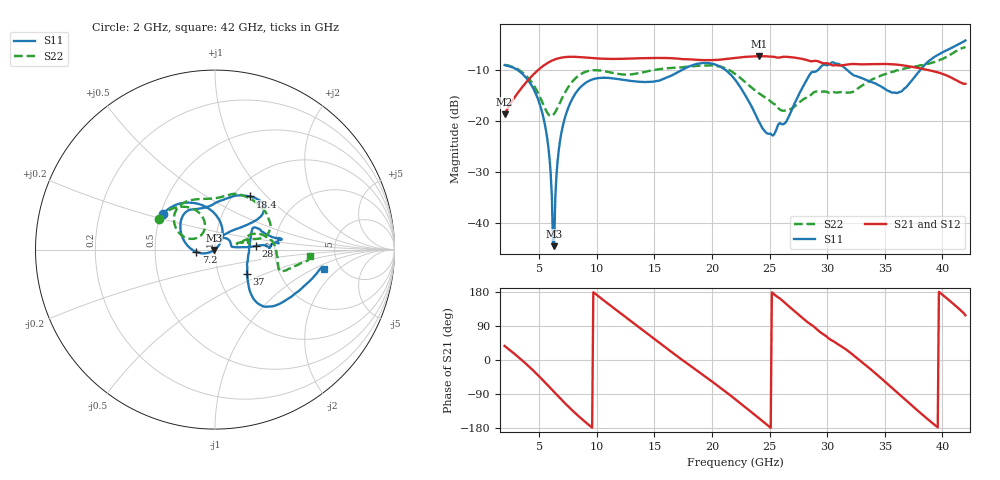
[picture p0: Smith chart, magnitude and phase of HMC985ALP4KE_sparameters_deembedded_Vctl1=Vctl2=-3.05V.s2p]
!s2p File: Measurements: S11, S21, S12, S22
# GHz S dB R 50.0
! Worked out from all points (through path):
!   401 points, 2 GHz to 42 GHz, reference 50 ohm
!   highest |S21| = -7.31 dB at 24.1 GHz (marker M1); lowest = -18.7 dB at 2 GHz (marker M2)
!   lowest |S11| = -44.5 dB at 6.3 GHz (marker M3), VSWR 1.01, Z = 49.5 - j0.26 ohm
!   |S11| at or under -10 dB: 3.122 GHz to 17.4 GHz (14.28 GHz wide, 139 % of centre); 21.17 GHz to 29.21 GHz (8.041 GHz wide, 31.9 % of centre); 31.73 GHz to 38.07 GHz (6.342 GHz wide, 18.2 % of centre)
!   |S22| runs from -19.0 to -5.5 dB; largest |S21 - S12| = 0.00051
!   S11 on the Smith chart (normalised r, x): 2 GHz: 0.51, +0.23; 7.2 GHz: 0.81, -0.02; 18.4 GHz: 1.19, +0.80; 28 GHz: 1.59, +0.07; 37 GHz: 1.37, -0.39; 42 GHz: 3.70, -1.31
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2  -9.06 145.7  -18.67 37.1  -18.67 37.1  -9.00 150.9
5  -16.35 78.2  -9.84 -43.3  -9.84 -43.3  -14.97 110.5
5.7  -23.44 56.5  -8.68 -65.3  -8.68 -65.3  -18.37 120.7
6.1  -34.72 46.3  -8.19 -78.2  -8.19 -78.2  -19.02 137.1
6.3  -44.55 -153.6  -8.00 -84.6  -8.00 -84.6  -18.59 145.2
6.7  -25.75 -157.5  -7.71 -97.4  -7.71 -97.4  -16.92 155.3
7.2  -19.65 -172.6  -7.50 -113.0  -7.50 -113.0  -14.60 157.7
8.7  -13.13 150.6  -7.51 -155.7  -7.51 -155.7  -10.71 141.6
12.4  -11.96 116.5  -7.81 115.7  -7.81 115.7  -10.91 96.0
15.4  -12.10 94.0  -7.66 46.3  -7.65 46.2  -9.85 73.5
18.4  -9.02 56.8  -7.98 -21.4  -7.98 -21.4  -9.27 56.3
22  -11.89 36.3  -7.63 -103.0  -7.64 -103.0  -10.76 14.9
24.1  -20.26 58.2  -7.31 -154.1  -7.31 -154.1  -14.63 17.6
25.4  -22.60 59.0  -7.43 173.3  -7.43 173.2  -16.67 14.4
28  -12.85 5.1  -7.92 107.2  -7.92 107.2  -15.66 13.6
28.7  -10.40 1.8  -8.29 91.5  -8.30 91.5  -14.65 12.5
30.5  -8.50 8.8  -9.11 50.1  -9.12 50.0  -14.40 14.8
32.4  -11.13 22.2  -8.84 9.6  -8.84 9.5  -14.07 22.1
35.4  -14.18 7.8  -8.86 -67.5  -8.85 -67.5  -10.57 13.8
37  -13.02 -36.9  -9.25 -110.7  -9.25 -110.7  -9.58 4.7
39.5  -7.21 -46.8  -10.41 -175.3  -10.41 -175.3  -8.28 -17.8
42  -4.22 -10.3  -12.71 118.0  -12.71 117.9  -5.50 -3.9
